FUNCTION FC 21 : VOID
TITLE =ANGLE AXIS ROTARY PRESS - VISUALISE
//
AUTHOR : Esposito
FAMILY : EGAL_srl
NAME : ANGLE_M
VERSION : 0.1


VAR_TEMP
  RETVAL : INT ;
  INMSR : BOOL ;
  RES_1 : BOOL ;
  RES_2 : BOOL ;
  RES_3 : BOOL ;
  RES_4 : BOOL ;
  RES_5 : BOOL ;
  RES_6 : BOOL ;
  RES_7 : BOOL ;
  RES_8 : BOOL ;
  RES_9 : BOOL ;
  RES_10 : BOOL ;
  RES_11 : BOOL ;
  RES_12 : BOOL ;
  RES_13 : BOOL ;
  RES_14 : BOOL ;
  RES_15 : BOOL ;
  DINT_RES : DINT ;
  WORD_RES : INT ;
  VALUES_AXIS : DINT ;
END_VAR
BEGIN
NETWORK
TITLE =CALL FC MSRMENT - READING ANGLE AXIS ROTARY PRESS

      CALL FC     7 (
           DB_NO                    := DB     1,
           RET_VAL                  := #RETVAL,
           IN_MSR                   := #INMSR);
      NOP   0;

NETWORK
TITLE =DIVISION - ACTUAL POSITION

      L     DB1.DBD   32;
      L     L#10000;
      /D    ;
      T     #VALUES_AXIS;
      NOP   0;
NETWORK
TITLE =VISUALIZE - ACTUAL POSITION

      L     #VALUES_AXIS;
      T     DB15.DBW    0;
      NOP   0;


END_FUNCTION

